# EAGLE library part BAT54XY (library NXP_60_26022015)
Schottky barrier quadruple diode in very small SOT363 package Schottky barrier quadruple diode with an integrated guard ring for stress protection. Two electrically isolated dual Schottky barrier diodes series, encapsulated in a SOT363 very small SMD plastic package. AAL Eindhoven MK
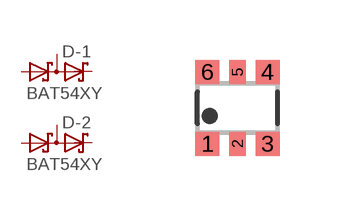
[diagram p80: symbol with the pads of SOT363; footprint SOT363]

Designator prefix D; gates -1=DIODE_SDD_AKAK -2=DIODE_SDD_AKAK

## BAT54XY  [SOT363]
1  -1:A1  pas
2  -1:K2  pas
3  -2:K1A2  pas
4  -2:A1  pas
5  -2:K2  pas
6  -1:K1A2  pas

## Footprint SOT363 (pad centres in mm)
SOT363 Plastic surface-mounted package; 6 leads JEDEC: -- IEC: -- JEITA: SC-88
smd 0.6 x 0.6: 1 -0.75,-0.9; 3 0.75,-0.9; 4 0.75,0.9; 6 -0.75,0.9
smd 0.4 x 0.6: 2 0,-0.9; 5 0,0.9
